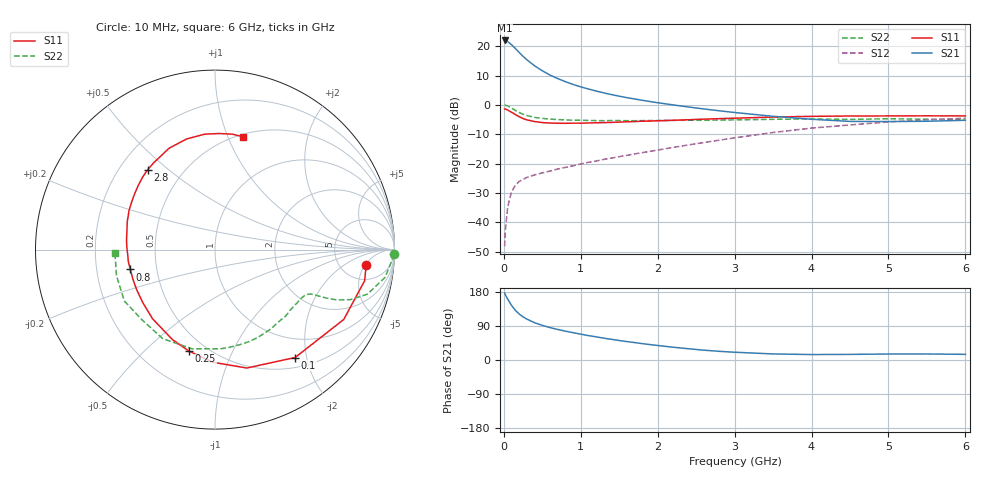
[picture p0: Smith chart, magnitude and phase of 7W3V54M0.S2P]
! Infineon Technologies  Discrete & RF Semiconductors
! BFS17W
! Si NPN RF Bipolar Junction Transistor in SOT323
! VCE = 3.5 V  IC = 4 mA
! Common Emitter S-Parameters:  August  1999
# GHz  S  MA  R  50
!  f  S11  S21  S12  S22
! GHz  MAG  ANG  MAG  ANG  MAG  ANG  MAG  ANG
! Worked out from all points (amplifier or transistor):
!   36 points, 10 MHz to 6 GHz, reference 50 ohm
!   highest |S21| = 22.0 dB at 10 MHz (marker M1)
!   |S21| within 3 dB of that: start of sweep to 159.2 MHz
!   unconditionally stable (mu >= 1): 607.7 MHz to 2.894 GHz; 4.21 GHz to end of sweep
!   at 250 MHz: K = 0.52, MSG = 21.0 dB, |S12| = -25.4 dB
!   at 1.4 GHz: K = 1.26, MAG = 7.7 dB, |S12| = -18.1 dB
!   at 6 GHz: K = 1.08, MAG = -2.1 dB, |S12| = -4.5 dB
!   S11 on the Smith chart (normalised r, x): 10 MHz: 9, -5; 100 MHz: 0.66, -1.80; 250 MHz: 0.40, -0.69; 800 MHz: 0.35, -0.10; 2.8 GHz: 0.32, +0.43; 6 GHz: 0.52, +1.13
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0.01  0.8471 -5.7  12.52 176.6  0.0039 86.4  0.9958 -1.5
0.02  0.8516 -11.8  12.46 172.1  0.0073 87.7  0.9854 -3.9
0.05  0.8161 -28.5  11.98 160.5  0.0181 76.5  0.9598 -9.3
0.1  0.7489 -53.4  10.6 144.2  0.0331 65.2  0.8849 -16.3
0.15  0.6831 -75.0  9.123 131.0  0.0427 55.6  0.8034 -20.3
0.2  0.6276 -91.1  7.811 121.3  0.0495 51.3  0.74 -22.3
0.25  0.5839 -104.3  6.715 113.8  0.0537 48.1  0.6912 -23.3
0.3  0.5549 -115.2  5.861 107.8  0.0579 46.8  0.6575 -23.8
0.4  0.5193 -132.0  4.632 98.4  0.064 46.2  0.6114 -24.4
0.5  0.499 -143.8  3.811 91.4  0.0692 47.3  0.5876 -24.9
0.6  0.4901 -153.3  3.221 85.6  0.0744 48.8  0.5712 -25.9
0.8  0.4846 -166.8  2.486 76.1  0.0859 52.2  0.5534 -28.9
0.9  0.4875 -172.1  2.228 72.1  0.0914 53.7  0.5472 -30.6
1.1  0.4912 178.6  1.861 64.4  0.1048 56.5  0.5425 -34.7
1.3  0.4988 170.6  1.6 57.6  0.1177 58.6  0.5374 -39.4
1.6  0.515 161.3  1.326 48.6  0.1376 61.3  0.5366 -46.8
2.2  0.5457 145.0  0.998 33.7  0.1882 64.8  0.5441 -63.4
2.8  0.5821 130.2  0.792 22.9  0.2498 64.7  0.5503 -81.4
3.5  0.6199 114.4  0.638 16.0  0.3379 60.6  0.5669 -103.0
4.5  0.6458 95.1  0.522 14.8  0.4545 48.8  0.5644 -136.1
5.5  0.6503 81.3  0.525 15.9  0.5535 36.2  0.5678 -165.2
6  0.6476 76.2  0.546 14.9  0.5926 30.0  0.5578 -178.0
